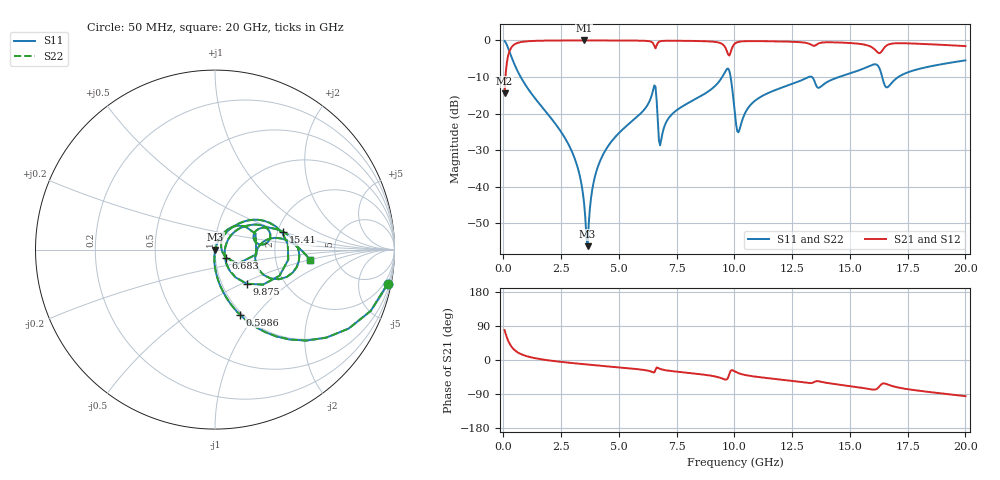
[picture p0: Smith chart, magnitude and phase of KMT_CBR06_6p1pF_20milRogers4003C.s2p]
! Data measured by Modelithics Inc. support@modelithics.com 813-866-6335
! KEMET CBR0603 6.1pF, Pad Width= 0.851mm, Pad Length= 0.64mm, Pad Gap= 0.62mm, 20mil Rogers 4003C substrate Data, January 2022
# hz S ma R 50
! 2 Port Network Data from SP1.SP block
! freq  magS11  angS11  magS21  angS21  magS12  angS12  magS22  angS22
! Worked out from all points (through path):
!   401 points, 50 MHz to 20 GHz, reference 50 ohm
!   highest |S21| = -0.01 dB at 3.491 GHz (marker M1); lowest = -14.4 dB at 50 MHz (marker M2)
!   group delay of S21, straight-line fit = 14.7 ps
!   lowest |S11| = -56.3 dB at 3.641 GHz (marker M3), VSWR 1.00, Z = 50.2 + j0.0295 ohm
!   |S11| at or under -10 dB: 744.5 MHz to 9.472 GHz (8.727 GHz wide, 171 % of centre); 9.835 GHz to 13.22 GHz (3.386 GHz wide, 29.4 % of centre); 13.35 GHz to 14.53 GHz (1.18 GHz wide, 8.46 % of centre)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
!   |S22| runs from -56.3 to -0.2 dB; largest |S21 - S12| = 0
!   S11 on the Smith chart (normalised r, x): 50 MHz: 1, -10; 598.6 MHz: 0.97, -0.83; 6.683 GHz: 1.13, -0.11; 9.875 GHz: 1.31, -0.53; 15.41 GHz: 2.14, +0.50; 20 GHz: 3.19, -0.53
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5e7  0.9818 -11.1  0.1899 78.9  0.1899 78.9  0.9818 -11.1
2.495e8  0.7178 -44.9  0.6957 45.1  0.6957 45.1  0.7178 -44.9
5.98625e8  0.3877 -69.1  0.9211 20.8  0.9211 20.8  0.3877 -69.1
2.74325e9  0.04172 -94.9  0.9978 -6.6  0.9978 -6.6  0.04172 -94.9
3.391625e9  0.01019 -92.9  0.9985 -10.5  0.9985 -10.5  0.01019 -92.9
3.491375e9  0.005914 -87.7  0.9985 -11.1  0.9985 -11.1  0.005914 -87.7
3.641e9  0.001531 11.1  0.9985 -12.0  0.9985 -12.0  0.001531 11.1
3.990125e9  0.01486 70.3  0.9983 -13.9  0.9983 -13.9  0.01486 70.3
4.488875e9  0.0342 70.6  0.9976 -16.6  0.9976 -16.6  0.0342 70.6
6.483875e9  0.2116 38.0  0.9094 -32.7  0.9094 -32.7  0.2116 38.0
6.683375e9  0.07782 -36.6  0.9247 -20.6  0.9247 -20.6  0.07782 -36.6
6.73325e9  0.04254 -16.6  0.9574 -22.2  0.9574 -22.2  0.04254 -16.6
9.376625e9  0.2847 35.8  0.9223 -46.8  0.9223 -46.8  0.2847 35.8
9.875375e9  0.2596 -47.1  0.7521 -26.8  0.7521 -26.8  0.2596 -47.1
1.0025e10  0.09734 -50.6  0.9076 -30.5  0.9076 -30.5  0.09734 -50.6
1.017462e10  0.05523 0.9  0.9542 -34.8  0.9542 -34.8  0.05523 0.9
1.10225e10  0.1604 41.9  0.9777 -44.8  0.9777 -44.8  0.1604 41.9
1.336662e10  0.3145 12.0  0.8585 -60.4  0.8585 -60.4  0.3145 12.0
1.54115e10  0.3919 14.6  0.8981 -72.3  0.8981 -72.3  0.3919 14.6
1.615962e10  0.466 -11.9  0.7062 -76.4  0.7062 -76.4  0.466 -11.9
1.670825e10  0.2408 2.9  0.8878 -66.2  0.8878 -66.2  0.2408 2.9
2e10  0.5332 -6.4  0.8356 -95.4  0.8356 -95.4  0.5332 -6.4
